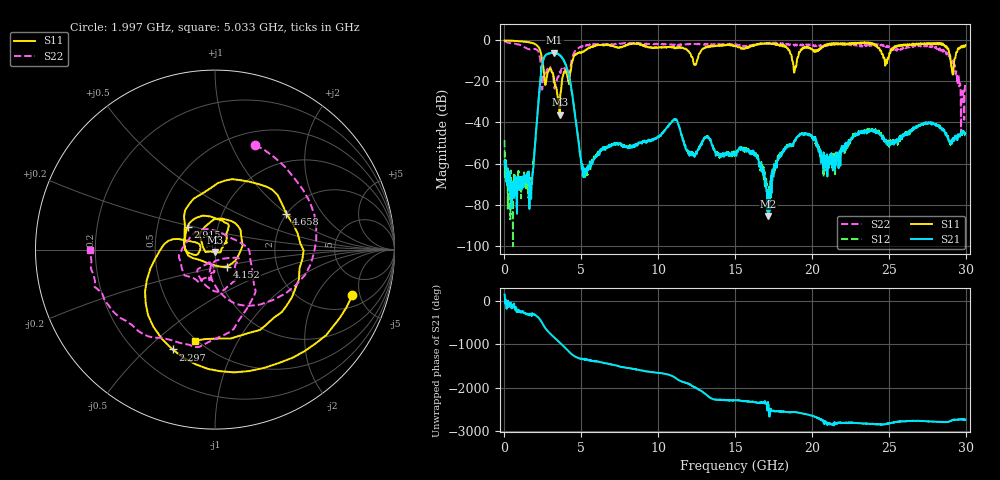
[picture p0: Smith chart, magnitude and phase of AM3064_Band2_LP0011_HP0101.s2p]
# Hz S DB R 50.0
!freq dBS11 angS11 dBS21 angS21 dBS12 angS12 dBS22 angS22
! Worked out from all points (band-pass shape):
!   1600 points, 10 MHz to 29.98 GHz, reference 50 ohm
!   highest |S21| = -5.97 dB at 3.234 GHz (marker M1); lowest = -85.6 dB at 17.16 GHz (marker M2)
!   |S21| within 3 dB of the highest: 2.549 GHz to 3.8 GHz (1.252 GHz wide, 39.4 % of centre)
!   lowest |S11| = -36.2 dB at 3.59 GHz (marker M3), VSWR 1.03, Z = 49.8 - j1.54 ohm
!   |S11| at or under -10 dB: 2.459 GHz to 4.428 GHz (1.97 GHz wide, 57.2 % of centre); 18.73 GHz to 19.02 GHz (294.7 MHz wide, 1.56 % of centre); 29.02 GHz to 29.25 GHz (228.1 MHz wide, 0.783 % of centre)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
!   |S22| runs from -45.2 to -0.2 dB; largest |S21 - S12| = 0.013
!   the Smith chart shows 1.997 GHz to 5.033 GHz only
!   S11 on the Smith chart (normalised r, x): 1.997 GHz: 2.90, -4.23; 2.297 GHz: 0.35, -0.61; 2.915 GHz: 0.71, +0.19; 4.152 GHz: 1.12, -0.22; 4.658 GHz: 1.99, +0.99; 5.033 GHz: 0.49, -0.68
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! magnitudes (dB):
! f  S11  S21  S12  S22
! 10 MHz  0.0  -58.6  -48.5  -0.2
! 366.1 MHz  -0.1  -65.3  -77.7  -1.3
! 1.603 GHz  -0.9  -67.1  -74.2  -4.3
! 1.997 GHz  -1.9  -50.0  -49.8  -4.1
! 2.297 GHz  -4.4  -22.4  -22.4  -8.1
! 2.915 GHz  -14.0  -6.4  -6.3  -12.6
! 3.234 GHz  -19.6  -6.0  -6.1  -22.6
! 3.59 GHz  -36.2  -7.2  -7.2  -15.2
! 4.152 GHz  -18.7  -15.9  -15.8  -19.7
! 4.658 GHz  -7.0  -39.9  -39.7  -5.0
! 5.015 GHz  -6.0  -60.7  -60.5  -3.2
! 5.033 GHz  -5.7  -62.9  -62.0  -3.1
! 10 GHz  -3.5  -46.8  -46.9  -1.8
! 15 GHz  -2.5  -55.3  -55.3  -1.9
! 16.32 GHz  -2.3  -55.7  -55.9  -2.1
! 17.16 GHz  -1.7  -85.6  -72.6  -1.4
! 18.19 GHz  -2.3  -54.1  -53.3  -1.8
! 19.99 GHz  -4.1  -46.3  -46.7  -2.1
! 20.87 GHz  -2.3  -61.9  -59.4  -2.8
! 25 GHz  -8.1  -50.4  -48.8  -2.8
! 28.56 GHz  -2.2  -43.2  -43.6  -4.6
! 29.98 GHz  -2.3  -45.5  -46.4  -21.7
